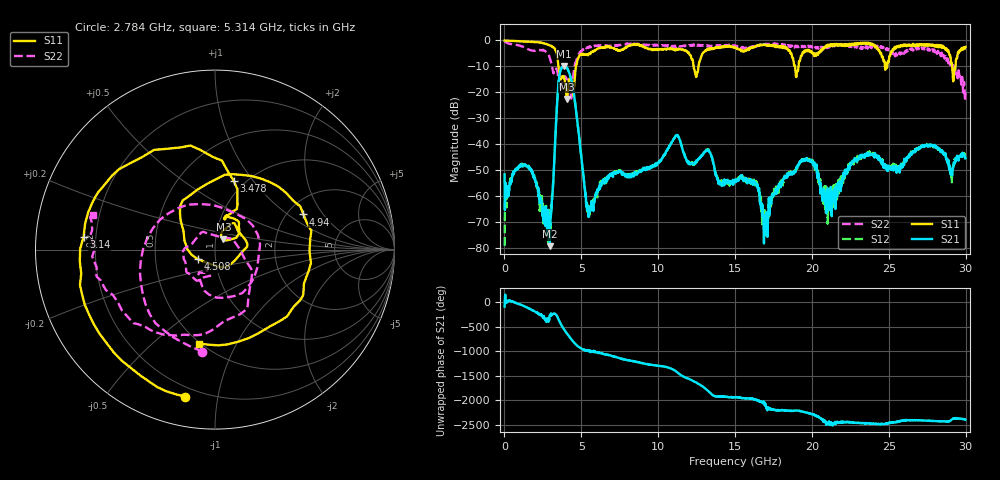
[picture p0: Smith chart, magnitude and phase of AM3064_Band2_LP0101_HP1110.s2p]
# Hz S DB R 50.0
!freq dBS11 angS11 dBS21 angS21 dBS12 angS12 dBS22 angS22
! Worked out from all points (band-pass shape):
!   1600 points, 10 MHz to 29.98 GHz, reference 50 ohm
!   highest |S21| = -9.85 dB at 3.89 GHz (marker M1); lowest = -79.2 dB at 2.953 GHz (marker M2)
!   |S21| within 3 dB of the highest: 3.592 GHz to 4.227 GHz (635 MHz wide, 16.2 % of centre)
!   lowest |S11| = -22.6 dB at 4.059 GHz (marker M3), VSWR 1.16, Z = 54.5 + j6.35 ohm
!   |S11| at or under -10 dB: 3.514 GHz to 4.645 GHz (1.131 GHz wide, 27.7 % of centre); 12.3 GHz to 12.63 GHz (320.2 MHz wide, 2.57 % of centre); 18.9 GHz to 19.13 GHz (230.6 MHz wide, 1.21 % of centre)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
!   |S22| runs from -23.3 to -0.2 dB; largest |S21 - S12| = 0.0085
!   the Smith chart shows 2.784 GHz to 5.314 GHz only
!   S11 on the Smith chart (normalised r, x): 2.784 GHz: 0.15, -0.81; 3.14 GHz: 0.15, +0.05; 3.478 GHz: 0.89, +0.81; 4.508 GHz: 0.82, -0.09; 4.94 GHz: 2.43, +1.32; 5.314 GHz: 0.49, -0.72
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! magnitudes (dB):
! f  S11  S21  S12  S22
! 10 MHz  0.0  -51.6  -79.1  -0.2
! 1.191 GHz  -0.4  -48.2  -47.5  -2.4
! 2.784 GHz  -1.6  -74.9  -68.1  -4.8
! 2.953 GHz  -2.0  -79.2  -67.3  -6.9
! 3.14 GHz  -2.7  -57.3  -57.4  -11.5
! 3.478 GHz  -8.1  -19.4  -19.3  -13.5
! 3.89 GHz  -14.7  -9.8  -10.0  -14.0
! 4.059 GHz  -22.6  -10.5  -10.5  -14.8
! 4.508 GHz  -19.2  -20.3  -20.3  -12.1
! 4.94 GHz  -5.5  -41.6  -41.8  -4.3
! 5.015 GHz  -5.6  -45.7  -45.8  -4.2
! 5.314 GHz  -5.5  -63.1  -63.5  -3.0
! 10 GHz  -3.5  -47.1  -47.2  -1.9
! 11.24 GHz  -3.6  -36.6  -36.6  -2.6
! 15 GHz  -2.7  -53.9  -54.6  -2.0
! 16.34 GHz  -2.3  -55.4  -55.0  -2.4
! 17.01 GHz  -1.8  -72.0  -70.8  -1.4
! 19.99 GHz  -4.4  -47.0  -46.5  -2.3
! 21.02 GHz  -1.8  -59.5  -70.6  -2.6
! 23.21 GHz  -1.3  -45.0  -45.4  -2.4
! 25 GHz  -8.0  -49.2  -48.5  -3.3
! 29.98 GHz  -2.6  -45.4  -45.0  -20.2
